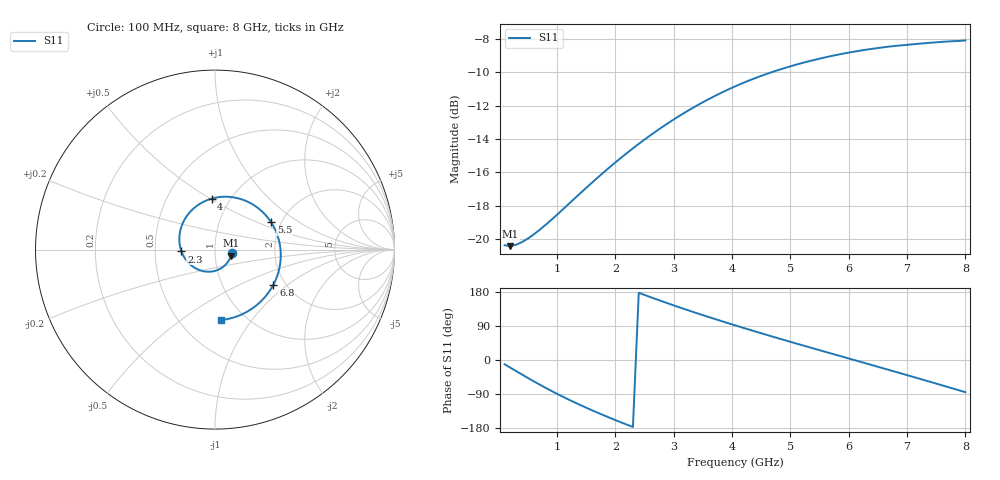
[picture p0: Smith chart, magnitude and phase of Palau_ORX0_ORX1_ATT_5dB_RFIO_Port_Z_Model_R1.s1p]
! Created Fri Oct  9 14:29:09 2020
! Palau ORX0/ORX1 RFIO Port Impedance Model.
! Attenuation  : 5 dB.
! Revision		: R1.
! Impedance Mode 	: Balanced Differential-Mode.
! Impedance Format 	: Series Equivalent Differential Impedance (SEDZ).
# hz S ma R 100
! 1 Port Network Data from SP1.SP block
! freq  magS11  angS11
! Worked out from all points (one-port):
!   80 points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, 100 MHz to 8 GHz, reference 100 ohm
!   lowest |S11| = -20.4 dB at 200 MHz (marker M1), VSWR 1.21, Z = 119 - j7.98 ohm
!   |S11| at or under -10 dB: start of sweep to 4.667 GHz
!   S11 on the Smith chart (normalised r, x): 100 MHz: 1.21, -0.05; 2.3 GHz: 0.69, -0.01; 4 GHz: 0.82, +0.51; 5.5 GHz: 1.78, +0.61; 6.8 GHz: 1.73, -0.80; 8 GHz: 0.78, -0.72
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1e8  0.09572 -11.4
2e8  0.09511 -20.4
6e8  0.1032 -56.3
9e8  0.1141 -81.4
1.1e9  0.1227 -97.0
1.3e9  0.1322 -111.9
1.6e9  0.1477 -132.8
2.1e9  0.1755 -164.8
2.3e9  0.1871 -176.8
2.7e9  0.2107 160.4
3.1e9  0.2343 138.8
3.5e9  0.2574 118.4
3.8e9  0.2739 103.6
4e9  0.2845 93.9
4.1e9  0.2896 89.2
4.4e9  0.3042 75.2
4.6e9  0.3133 66.0
4.8e9  0.3219 56.9
5.1e9  0.3337 43.5
5.5e9  0.3478 25.9
5.8e9  0.3572 12.8
6.1e9  0.3653 -0.4
6.4e9  0.3723 -13.5
6.8e9  0.3799 -31.1
7.1e9  0.3842 -44.4
7.4e9  0.3882 -57.8
7.6e9  0.3907 -66.8
8e9  0.3945 -85.0
